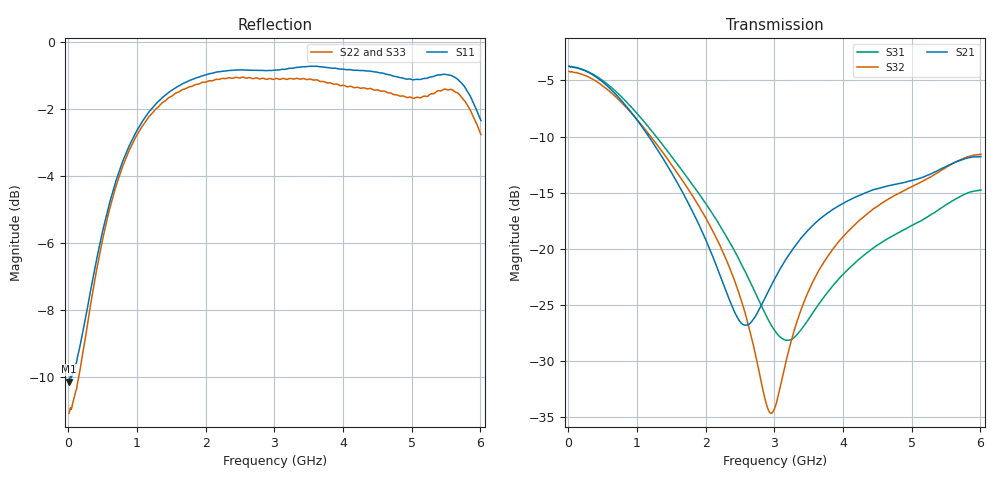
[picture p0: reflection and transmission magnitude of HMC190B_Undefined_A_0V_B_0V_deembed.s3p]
! Device:	HMC190B
! Description:	GaAs MMIC SPDT Reflective Switch
! Package:	8-lead mini small outline package
! Frequency:	DC -  3 GHz
! Ports:
! RFC = Port 1
! RF1 = Port 2
! RF2 = Port 3
! State: Undefined
! Control Voltages:
! A  = 0 V
! B  = 0 V
! Data:	Data was collected using a calibrated network analyzer with AFR software.
!	Fixtures were calculated using AFR and fixturing was applied to collect
!	this Deembedded  S Parameter data of HMC190B.
! Note:	Analog Devices supplies this data as a sample of measured data at the package pin
!	for this product.  Your particular data for this product may vary.
!	Data was taken at 25 degrees C.
!	Analog Devices reserves the right to change this data at anytime.
# Hz S  dB  R 50
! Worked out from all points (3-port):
!   601 points, 10 MHz to 6.01 GHz, reference 50 ohm
!   strongest paths, dB at 10 MHz, 1.51 GHz, 3.01 GHz, 4.51 GHz, 6.01 GHz:
!     S21: -3.7, -13.3, -22.6, -14.6, -11.8
!     S32: -4.2, -12.6, -34.1, -16.2, -11.6
!     S31: -3.7, -11.8, -27.3, -19.6, -14.8
!   lowest |S11| = -10.1 dB at 10 MHz (marker M1), VSWR 1.91, Z = 26.2 - j0.498 ohm
!   |S11| at or under -10 dB: start of sweep to 23.46 MHz; 36.97 MHz to 42.91 MHz (5.938 MHz wide, 14.9 % of centre)
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1e7  -10.13 -178.4  -3.73 -1.2  -3.72 -1.1
     -3.72 -1.2  -11.07 -177.9  -4.19 -1.2
     -3.73 -1.1  -4.19 -1.2  -11.04 -178.0
6.1e8  -4.72 -167.2  -5.73 -45.6  -5.54 -46.4
       -5.73 -45.6  -4.90 -162.8  -6.03 -48.6
       -5.54 -46.4  -6.02 -48.6  -5.02 -162.1
1.38e9  -1.63 163.7  -11.96 -82.8  -10.78 -85.9
        -11.97 -82.8  -1.79 168.2  -11.47 -93.0
        -10.78 -86.0  -11.45 -93.0  -1.84 170.4
2.51e9  -0.83 130.1  -26.58 -56.7  -21.23 -106.1
        -26.56 -56.7  -1.06 134.2  -24.48 -144.7
        -21.24 -106.2  -24.43 -144.8  -1.05 138.7
2.89e9  -0.85 119.4  -24.06 -11.4  -26.01 -92.2
        -24.05 -11.4  -1.11 123.7  -34.07 155.4
        -26.06 -92.5  -33.95 156.3  -1.07 129.4
3.01e9  -0.83 116.0  -22.63 -6.2  -27.26 -81.6
        -22.63 -6.3  -1.09 120.2  -34.14 108.5
        -27.31 -81.8  -34.12 109.7  -1.07 126.5
3.43e9  -0.73 104.6  -18.75 -3.2  -26.83 -37.9
        -18.76 -3.2  -1.09 108.9  -24.74 46.2
        -26.88 -37.7  -24.78 46.5  -1.08 116.7
3.94e9  -0.80 91.4  -16.16 -11.1  -22.66 -22.9
        -16.16 -11.1  -1.28 95.1  -19.33 22.2
        -22.67 -22.7  -19.34 22.4  -1.21 105.0
5.27e9  -1.04 65.4  -13.35 -32.5  -17.00 -36.4
        -13.35 -32.5  -1.55 69.0  -13.63 -16.9
        -17.00 -36.3  -13.62 -16.8  -1.49 77.3
6.01e9  -2.33 62.0  -11.77 -34.5  -14.76 -41.4
        -11.77 -34.5  -2.75 66.2  -11.57 -25.2
        -14.76 -41.5  -11.56 -25.2  -2.83 69.4
